| IBIS file imx8dxl_15x15_rev1_15.ibs generated by Viper version: 2018.06.11
[IBIS Ver]   5.1
[Comment Char]   |_char
[File Name]   imx8dxl_15x15_rev1_15.ibs
[File Rev]   1.15
[Date]   Mon Sep  2 11:08:28 2019
[Source]   NXP Viper 2018.06.11
[Notes]
   Warning 'pullup_ref' Exceeds 15 characters: VDD_PCIE_DIG_1P8_3P3 was cut to VDD_PCIE_DIG_1P
   Warning 'pullup_ref' Exceeds 15 characters: VDD_PCIE_LDO_1P0_CAP was cut to VDD_PCIE_LDO_1P
   Warning 'pullup_ref' Exceeds 15 characters: VDD_EMMC0_1P8_3P3 was cut to VDD_EMMC0_1P8_3
   Warning 'pullup_ref' Exceeds 15 characters: VDD_USDHC1_VSELECT_1P8_3P3 was cut to VDD_USDHC1_VSEL
   Warning 'pullup_ref' Exceeds 15 characters: VDD_ENET0_1P8_3P3 was cut to VDD_ENET0_1P8_3
   Warning 'pullup_ref' Exceeds 15 characters: VDD_ENET0_VSELECT_1P8_3P3 was cut to VDD_ENET0_VSELE
   Warning 'pullup_ref' Exceeds 15 characters: VDD_ENET_MDIO_1P8_3P3 was cut to VDD_ENET_MDIO_1
   Warning 'pullup_ref' Exceeds 15 characters: VDD_ESAI_SPDIF_1P8_3P3 was cut to VDD_ESAI_SPDIF_
   Warning 'pullup_ref' Exceeds 15 characters: VDD_SPI_MCLK_UART_1P8_3P3 was cut to VDD_SPI_MCLK_UA
   Warning 'pullup_ref' Exceeds 15 characters: VDD_SPI_SAI_1P8_3P3 was cut to VDD_SPI_SAI_1P8
   Warning 'pullup_ref' Exceeds 15 characters: VDD_QSPI0B_1P8_3P3 was cut to VDD_QSPI0B_1P8_
   Warning 'pullup_ref' Exceeds 15 characters: VDD_QSPI0A_1P8_3P3 was cut to VDD_QSPI0A_1P8_
   Warning 'pullup_ref' Exceeds 15 characters: VDD_TMPR_CSI_1P8_3P3 was cut to VDD_TMPR_CSI_1P
   Warning 'pullup_ref' Exceeds 15 characters: VDD_SNVS_LDO_1P8_CAP was cut to VDD_SNVS_LDO_1P
   Warning 'pullup_ref' Exceeds 15 characters: VDD_CAN_UART_1P8_3P3 was cut to VDD_CAN_UART_1P
[Disclaimer] IMPORTANT NOTICE
  This information is provided on an AS IS basis and without warranty.
  IN NO EVENT SHALL NXP BE LIABLE FOR INCIDENTAL OR CONSEQUENTIAL
  DAMAGES ARISING FROM USE OF THIS INFORMATION. THIS DISCLAIMER OF
  WARRANTY EXTENDS TO THE USER OF THE INFORMATION, AND TO THEIR CUSTOMERS
  OR USERS OF PRODUCTS  AND IS IN LIEU OF ALL WARRANTIES WHETHER EXPRESS,
  IMPLIED, OR STATUTORY, INCLUDING IMPLIED WARRANTIES OF MERCHANTABILITY
  OR FITNESS FOR PARTICULAR PURPOSE.
  NXP does not represent or warrant that the information furnished
  hereunder is free of infringement of any third party patents,
  copyrights, trade secrets, or other intellectual property rights.
  NXP does not represent or warrant that the information is free of
  defect, or that it meets any particular standard, requirements or need
  of the user of the infomation or their customers.
  NXP reserves the right to change the information in this file
  without notice.
   http://www.nxp.com
[Copyright]   (C) Copyright NXP 2004 - 2019, All Rights Reserved.
|   15x15
[Component]   15x15
[Manufacturer]   NXP
[Package]
| variable   typ   min   max
R_pkg   0.39888   0.071395   0.70153
L_pkg   2.436e-09   7.469e-10   4.204e-09
C_pkg   1.081e-12   6.841e-13   1.885e-12
[Pin] signal_name   model_name   R_pin   L_pin   C_pin
A1   VSS_MAIN   GND   NA   NA   NA
A3   DDR_DCF22   PDDRIO_PAD_COMMAND   0.69334   4.204e-09 1.534e-12
A5   DDR_DCF09   PDDRIO_PAD_COMMAND   0.65039   4.090e-09 1.750e-12
A7   DDR_DCF04   PDDRIO_PAD_COMMAND   0.70153   4.051e-09 1.549e-12
A9   PCIE_CTRL0_WAKE_B   BDPROGSCARUDQP_SDMMC_STD_3V3SF_FC_OUTER  0.37798   2.410e-09 9.804e-13
A11   PCIE0_TX0_P   ABI_SERDES   0.33546   2.531e-09 1.007e-12
A13   PCIE0_RX0_P   ABI_SERDES   0.33039   2.526e-09 1.001e-12
A15   PCIE_REFCLK100M_P   NC   0.39132   2.612e-09 9.561e-13
A17   USB_OTG2_DP   USB2_NXP   0.36476   2.455e-09 9.409e-13
A19   USB_OTG1_DN   USB2_NXP   0.3104   2.238e-09 9.070e-13
A21   EMMC0_DATA7   BDPROGSCARUDQP_SDMMC_STD_3V3SF_FC_OUTER  0.50159   3.076e-09 1.290e-12
A23   EMMC0_DATA0   BDPROGSCARUDQP_SDMMC_STD_3V3SF_FC_INNER  0.39707   2.449e-09 1.054e-12
A25   EMMC0_DATA5   BDPROGSCARUDQP_SDMMC_STD_3V3SF_FC_OUTER  0.39485   2.459e-09 1.043e-12
A27   EMMC0_CMD   BDPROGSCARUDQP_SDMMC_STD_3V3SF_FC_OUTER  0.47205   2.883e-09 1.198e-12
A29   USDHC1_RESET_B   BDPROGSCARUDQP_SDMMC_STD_3V3SF_FC_INNER  0.43085   2.711e-09 1.176e-12
A31   ENET0_RGMII_RXD3   BDPROGSCARUDQP_SDMMC_STD_3V3SF_FC_OUTER  0.5841   3.378e-09 1.362e-12
A33   ENET0_RGMII_RXD1   BDPROGSCARUDQP_SDMMC_STD_3V3SF_FC_OUTER  0.49079   2.887e-09 1.171e-12
A35   VSS_MAIN   GND   NA   NA   NA
B2   DDR_DCF20   PDDRIO_PAD_COMMAND   0.63836   3.791e-09 1.427e-12
B4   DDR_DCF17   PDDRIO_PAD_COMMAND   0.58041   3.372e-09 1.383e-12
B6   DDR_DCF19   PDDRIO_PAD_COMMAND   0.63149   3.649e-09 1.445e-12
B8   PCIE_CTRL0_PERST_B   BDPROGSCARUDQP_SDMMC_STD_3V3SF_FC_OUTER  0.32639   2.064e-09 1.009e-12
B10   PCIE0_TX0_N   ABI_SERDES   0.34946   2.450e-09 1.035e-12
B12   PCIE0_RX0_N   ABI_SERDES   0.33887   2.428e-09 1.004e-12
B14   PCIE_REFCLK100M_N   NC   0.39474   2.595e-09 9.576e-13
B16   USB_OTG2_DN   USB2_NXP   0.35865   2.350e-09 9.326e-13
B18   USB_OTG1_DP   USB2_NXP   0.32362   2.267e-09 9.280e-13
B20   EMMC0_DATA6   BDPROGSCARUDQP_SDMMC_STD_3V3SF_FC_INNER  0.34554   2.183e-09 9.968e-13
B22   EMMC0_DATA1   BDPROGSCARUDQP_SDMMC_STD_3V3SF_FC_OUTER  0.31728   1.984e-09 9.313e-13
B24   EMMC0_DATA3   BDPROGSCARUDQP_SDMMC_STD_3V3SF_FC_OUTER  0.32903   2.044e-09 9.577e-13
B26   EMMC0_RESET_B   BDPROGSCARUDQP_SDMMC_STD_3V3SF_FC_OUTER  0.37344   2.349e-09 1.036e-12
B28   USDHC1_VSELECT   BDPROGSCARUDQP_SDMMC_STD_3V3SF_FC_OUTER  0.43171   2.674e-09 1.183e-12
B30   USDHC1_WP   BDPROGSCARUDQP_SDMMC_STD_3V3SF_FC_INNER  0.43147   2.643e-09 1.163e-12
B32   ENET0_RGMII_RXD0   BDPROGSCARUDQP_SDMMC_STD_3V3SF_FC_INNER  0.49885   2.934e-09 1.197e-12
B34   ENET0_RGMII_RXC   BDPROGSCARUDQP_SDMMC_STD_3V3SF_FC_INNER  0.52236   3.036e-09 1.292e-12
C1   VSS_MAIN   GND   NA   NA   NA
C3   VSS_MAIN   GND   NA   NA   NA
C5   DDR_DCF32   PDDRIO_PAD_COMMAND   0.42657   2.729e-09 1.182e-12
C7   VSS_MAIN   GND   NA   NA   NA
C9   PCIE_CTRL0_CLKREQ_B   BDPROGSCARUDQP_SDMMC_STD_3V3SF_FC_INNER  0.31061   1.972e-09 8.875e-13
C11   VSS_MAIN   GND   NA   NA   NA
C13   VSS_MAIN   GND   NA   NA   NA
C15   VSS_MAIN   GND   NA   NA   NA
C17   VSS_MAIN   GND   NA   NA   NA
C19   USB_OTG1_ID   NC   0.32886   2.060e-09 9.688e-13
C21   EMMC0_DATA2   BDPROGSCARUDQP_SDMMC_STD_3V3SF_FC_INNER  0.28685   1.796e-09 8.761e-13
C23   EMMC0_DATA4   BDPROGSCARUDQP_SDMMC_STD_3V3SF_FC_INNER  0.28187   1.779e-09 8.664e-13
C25   EMMC0_STROBE   BDPROGSCARUDQP_SDMMC_STD_3V3SF_FC_INNER  0.33656   2.067e-09 9.738e-13
C27   EMMC0_CLK   BDPROGSCARUDQP_SDMMC_STD_3V3SF_FC_INNER  0.52053   3.084e-09 1.318e-12
C29   USDHC1_CD_B   BDPROGSCARUDQP_SDMMC_STD_3V3SF_FC_OUTER  0.42428   2.608e-09 1.152e-12
C31   ENET0_RGMII_RXD2   BDPROGSCARUDQP_SDMMC_STD_3V3SF_FC_INNER  0.52682   3.001e-09 1.274e-12
C33   ENET0_RGMII_RX_CTL   BDPROGSCARUDQP_SDMMC_STD_3V3SF_FC_OUTER  0.42005   2.537e-09 1.127e-12
C35   ENET0_RGMII_TX_CTL   BDPROGSCARUDQP_SDMMC_STD_3V3SF_FC_OUTER  0.51478   3.058e-09 1.280e-12
D2   VSS_MAIN   GND   NA   NA   NA
D34   ENET0_REFCLK_125M_25M   BDPROGSCARUDQP_SDMMC_STD_3V3SF_FC_OUTER  0.45684   2.681e-09 1.102e-12
E1   DDR_DCF24   PDDRIO_PAD_COMMAND   0.6095   3.695e-09 1.338e-12
E3   DDR_DCF27   PDDRIO_PAD_COMMAND   0.43126   2.639e-09 1.204e-12
E5   VSS_MAIN   GND   NA   NA   NA
E7   VSS_MAIN   GND   NA   NA   NA
E9   VSS_MAIN   GND   NA   NA   NA
E11   VDD_PCIE_LDO_1P0_CAP   POWER   NA   NA   NA
E13   VSS_MAIN   GND   NA   NA   NA
E15   VDD_ANA0_1P8   POWER   NA   NA   NA
E17   VSS_MAIN   GND   NA   NA   NA
E19   VSS_MAIN   GND   NA   NA   NA
E21   VSS_MAIN   GND   NA   NA   NA
E23   VSS_MAIN   GND   NA   NA   NA
E25   VSS_MAIN   GND   NA   NA   NA
E27   VSS_MAIN   GND   NA   NA   NA
E29   VSS_MAIN   GND   NA   NA   NA
E31   VSS_MAIN   GND   NA   NA   NA
E33   ENET0_MDC   BDPROGSCARUDQP_SDMMC_STD_3V3SF_FC_OUTER  0.39205   2.311e-09 1.041e-12
E35   ENET0_MDIO   BDPROGSCARUDQP_SDMMC_STD_3V3SF_FC_INNER  0.47347   2.857e-09 1.148e-12
F2   DDR_DCF23   PDDRIO_PAD_COMMAND   0.51126   3.016e-09 1.214e-12
F34   ENET1_RGMII_RXD1   BDPROGSCARUDQP_SDMMC_STD_3V3SF_FC_OUTER  0.46877   2.793e-09 1.175e-12
G1   DDR_DCF26   PDDRIO_PAD_COMMAND   0.5185   3.175e-09 1.322e-12
G3   VSS_MAIN   GND   NA   NA   NA
G5   VSS_MAIN   GND   NA   NA   NA
G9   PCIE_REXT   NC   0.34925   2.509e-09 1.529e-12
G11   PCIE_REF_QR   NC   0.23973   1.816e-09 9.243e-13
G13   USB_OTG2_VBUS   hs_vbus_input   0.21475   1.509e-09 7.043e-13
G15   USB_OTG2_ID   NC   0.21462   1.402e-09 7.583e-13
G17   USB_OTG1_VBUS   hs_vbus_input   0.24172   1.565e-09 7.717e-13
G19   USB_SS3_TC1   BDPROGSCARUDQP_SDMMC_STD_3V3SF_FC_OUTER  0.19904   1.304e-09 6.960e-13
G21   USB_SS3_TC0   BDPROGSCARUDQP_SDMMC_STD_3V3SF_FC_INNER  0.30844   1.974e-09 9.084e-13
G23   USB_SS3_TC3   BDPROGSCARUDQP_SDMMC_STD_3V3SF_FC_OUTER  0.29844   1.856e-09 9.049e-13
G25   USB_SS3_TC2   BDPROGSCARUDQP_SDMMC_STD_3V3SF_FC_INNER  0.40848   2.503e-09 1.109e-12
G27   ENET0_RGMII_TXC   BDPROGSCARUDQP_SDMMC_STD_3V3SF_FC_INNER  0.24271   1.576e-09 8.194e-13
G29   ENET0_RGMII_TXD1   BDPROGSCARUDQP_SDMMC_STD_3V3SF_FC_OUTER  0.3428   2.080e-09 9.846e-13
G31   VSS_MAIN   GND   NA   NA   NA
G33   ENET1_RGMII_RXC   BDPROGSCARUDQP_SDMMC_STD_3V3SF_FC_INNER  0.39056   2.383e-09 1.023e-12
G35   ENET1_RGMII_RXD3   BDPROGSCARUDQP_SDMMC_STD_3V3SF_FC_OUTER  0.44701   2.719e-09 1.173e-12
H2   DDR_DCF18   PCKE_PAD   0.49331   2.908e-09 1.114e-12
H34   ENET1_RGMII_RXD2   BDPROGSCARUDQP_SDMMC_STD_3V3SF_FC_INNER  0.40015   2.450e-09 1.063e-12
J1   DDR_DCF01   PDDRIO_PAD_COMMAND   0.54249   3.171e-09 1.259e-12
J3   DDR_DCF03   PDDRIO_PAD_COMMAND   0.49918   2.845e-09 1.237e-12
J5   VSS_MAIN   GND   NA   NA   NA
J7   DDR_DCF28   PDDRIO_PAD_COMMAND   0.27786   1.824e-09 8.557e-13
J9   DDR_DCF33   PDDRIO_PAD_COMMAND   0.37754   2.473e-09 1.129e-12
J11   PCIE0_PHY_PLL_REF_RETURN   GND   0.071395  7.469e-10 1.106e-12
J13   VDD_PCIE_1P8   POWER   NA   NA   NA
J17   VDD_USB_SS3_LDO_1P0_CAP   POWER   NA   NA   NA
J19   VDD_USB_1P8   POWER   NA   NA   NA
J21   VDD_USB_3P3   POWER   NA   NA   NA
J23   VDD_EMMC0_1P8_3P3   POWER   NA   NA   NA
J25   VDD_EMMC0_1P8_3P3   POWER   NA   NA   NA
J27   VDD_USDHC1_VSELECT_1P8_3P3   POWER   NA   NA   NA
J29   ENET0_RGMII_TXD0   BDPROGSCARUDQP_SDMMC_STD_3V3SF_FC_INNER  0.36245   2.190e-09 9.561e-13
J31   VSS_MAIN   GND   NA   NA   NA
J33   ENET1_RGMII_RXD0   BDPROGSCARUDQP_SDMMC_STD_3V3SF_FC_INNER  0.39699   2.409e-09 1.053e-12
J35   ENET1_RGMII_RX_CTL   BDPROGSCARUDQP_SDMMC_STD_3V3SF_FC_OUTER  0.46113   2.750e-09 1.160e-12
K2   DDR_CK0_N   PCK_PAD   0.59967   3.394e-09 1.352e-12
K34   ENET1_REFCLK_125M_25M   BDPROGSCARUDQP_SDMMC_STD_3V3SF_FC_OUTER  0.40652   2.458e-09 1.069e-12
L1   DDR_CK0_P   PCK_PAD   0.58582   3.373e-09 1.364e-12
L3   VSS_MAIN   GND   NA   NA   NA
L5   VSS_MAIN   GND   NA   NA   NA
L7   DDR_DCF30   PCKE_PAD   0.27406   1.691e-09 8.614e-13
L9   VDD_PCIE_DIG_1P8_3P3   POWER   NA   NA   NA
L11   VSS_MAIN   GND   NA   NA   NA
L13   VSS_MAIN   GND   NA   NA   NA
L15   VSS_MAIN   GND   NA   NA   NA
L17   VSS_MAIN   GND   NA   NA   NA
L19   VSS_MAIN   GND   NA   NA   NA
L21   VSS_MAIN   GND   NA   NA   NA
L23   VSS_MAIN   GND   NA   NA   NA
L25   VSS_MAIN   GND   NA   NA   NA
L27   VDD_ENET0_VSELECT_1P8_3P3   POWER   NA   NA   NA
L29   ENET0_RGMII_TXD2   BDPROGSCARUDQP_SDMMC_STD_3V3SF_FC_INNER  0.3233   2.047e-09 9.997e-13
L31   VSS_MAIN   GND   NA   NA   NA
L33   ENET1_RGMII_TXD3   BDPROGSCARUDQP_SDMMC_STD_3V3SF_FC_OUTER  0.35635   2.156e-09 9.575e-13
L35   ENET1_RGMII_TXC   BDPROGSCARUDQP_SDMMC_STD_3V3SF_FC_INNER  0.5103   3.102e-09 1.230e-12
M2   DDR_DCF05   PDDRIO_PAD_COMMAND   0.3749   2.205e-09 9.777e-13
M34   ENET1_RGMII_TXD2   BDPROGSCARUDQP_SDMMC_STD_3V3SF_FC_OUTER  0.52172   3.043e-09 1.266e-12
N1   DDR_DCF00   PDDRIO_PAD_COMMAND   0.39316   2.320e-09 1.064e-12
N3   DDR_DCF08   PDDRIO_PAD_COMMAND   0.51713   2.935e-09 1.237e-12
N5   VSS_MAIN   GND   NA   NA   NA
N7   VDD_DDR_VDDQ   POWER   NA   NA   NA
N9   VDD_DDR_VDDQ   POWER   NA   NA   NA
N11   VSS_MAIN   GND   NA   NA   NA
N13   VDD_MEMC   POWER   NA   NA   NA
N15   VDD_MAIN   POWER   NA   NA   NA
N17   VDD_MAIN   POWER   NA   NA   NA
N19   VDD_MAIN   POWER   NA   NA   NA
N21   VDD_MAIN   POWER   NA   NA   NA
N23   VDD_MAIN   POWER   NA   NA   NA
N25   VSS_MAIN   GND   NA   NA   NA
N27   VDD_ENET0_1P8_3P3   POWER   NA   NA   NA
N29   ENET0_RGMII_TXD3   BDPROGSCARUDQP_SDMMC_STD_3V3SF_FC_OUTER  0.33799   2.054e-09 9.689e-13
N31   VSS_MAIN   GND   NA   NA   NA
N33   ENET1_RGMII_TXD0   BDPROGSCARUDQP_SDMMC_STD_3V3SF_FC_INNER  0.37304   2.268e-09 1.025e-12
N35   ENET1_RGMII_TXD1   BDPROGSCARUDQP_SDMMC_STD_3V3SF_FC_OUTER  0.43036   2.644e-09 1.159e-12
P2   DDR_DCF15   PCKE_PAD   0.44408   2.646e-09 1.078e-12
P34   SPI3_SCK   BDPROGSCARUDQP_SDMMC_STD_3V3SF_FC_INNER  0.34281   2.124e-09 9.884e-13
R1   DDR_DCF10   PDDRIO_PAD_COMMAND   0.47803   2.820e-09 1.199e-12
R3   VSS_MAIN   GND   NA   NA   NA
R5   VSS_MAIN   GND   NA   NA   NA
R7   VDD_DDR_VDDQ   POWER   NA   NA   NA
R9   VDD_DDR_VDDQ   POWER   NA   NA   NA
R11   VSS_MAIN   GND   NA   NA   NA
R13   VDD_MEMC   POWER   NA   NA   NA
R15   VDD_MAIN   POWER   NA   NA   NA
R17   VDD_MAIN   POWER   NA   NA   NA
R19   VSS_MAIN   GND   NA   NA   NA
R21   VSS_MAIN   GND   NA   NA   NA
R23   VDD_MAIN   POWER   NA   NA   NA
R25   VSS_MAIN   GND   NA   NA   NA
R27   VDD_ENET_MDIO_1P8_3P3   POWER   NA   NA   NA
R29   ENET1_RGMII_TX_CTL   BDPROGSCARUDQP_SDMMC_STD_3V3SF_FC_INNER  0.40442   2.374e-09 1.066e-12
R31   VSS_MAIN   GND   NA   NA   NA
R33   SPI3_SDI   BDPROGSCARUDQP_SDMMC_STD_3V3SF_FC_INNER  0.34862   2.106e-09 9.636e-13
R35   SPI3_SDO   BDPROGSCARUDQP_SDMMC_STD_3V3SF_FC_OUTER  0.41808   2.511e-09 1.122e-12
T2   DDR_DCF14   PCKE_PAD   0.41078   2.375e-09 9.867e-13
T34   SPI3_CS0   BDPROGSCARUDQP_SDMMC_STD_3V3SF_FC_OUTER  0.36788   2.237e-09 1.022e-12
U1   DDR_DCF16   PDDRIO_PAD_COMMAND   0.37334   2.217e-09 8.753e-13
U3   DDR_DCF12   PDDRIO_PAD_COMMAND   0.37509   2.173e-09 9.658e-13
U5   VSS_MAIN   GND   NA   NA   NA
U7   VDD_DDR_VDDQ   POWER   NA   NA   NA
U9   VDD_DDR_VDDQ   POWER   NA   NA   NA
U11   VSS_MAIN   GND   NA   NA   NA
U13   VDD_MEMC   POWER   NA   NA   NA
U15   VSS_MAIN   GND   NA   NA   NA
U17   VSS_MAIN   GND   NA   NA   NA
U19   VDD_MEMC   POWER   NA   NA   NA
U21   VSS_MAIN   GND   NA   NA   NA
U23   VDD_MAIN   POWER   NA   NA   NA
U25   VSS_MAIN   GND   NA   NA   NA
U27   VDD_ESAI_SPDIF_1P8_3P3   POWER   NA   NA   NA
U29   SPI3_CS1   BDPROGSCARUDQP_SDMMC_STD_3V3SF_FC_INNER  0.27919   1.718e-09 8.422e-13
U31   VSS_MAIN   GND   NA   NA   NA
U33   MCLK_IN0   BDPROGSCARUDQP_SDMMC_STD_3V3SF_FC_INNER  0.28929   1.788e-09 8.790e-13
U35   MCLK_IN1   BDPROGSCARUDQP_SDMMC_STD_3V3SF_FC_OUTER  0.37626   2.307e-09 1.050e-12
V2   DDR_DCF21   PDDRIO_PAD_COMMAND   0.48159   2.850e-09 1.140e-12
V34   MCLK_OUT0   BDPROGSCARUDQP_SDMMC_STD_3V3SF_FC_OUTER  0.36526   2.211e-09 9.998e-13
W1   DDR_DCF11   PDDRIO_PAD_COMMAND   0.40855   2.365e-09 9.927e-13
W3   VSS_MAIN   GND   NA   NA   NA
W5   VSS_MAIN   GND   NA   NA   NA
W7   VDD_DDR_PLL_1P8   POWER   NA   NA   NA
W9   VDD_DDR_VDDQ   POWER   NA   NA   NA
W11   VSS_MAIN   GND   NA   NA   NA
W13   VDD_MEMC   POWER   NA   NA   NA
W15   VDD_MEMC   POWER   NA   NA   NA
W17   VDD_MEMC   POWER   NA   NA   NA
W19   VDD_MEMC   POWER   NA   NA   NA
W21   VSS_MAIN   GND   NA   NA   NA
W23   VDD_MAIN   POWER   NA   NA   NA
W25   VSS_MAIN   GND   NA   NA   NA
W27   VDD_SPI_MCLK_UART_1P8_3P3   POWER   NA   NA   NA
W29   UART1_RTS_B   BDPROGSCARUDQP_SDMMC_STD_3V3SF_FC_INNER  0.1996   1.313e-09 6.989e-13
W31   VSS_MAIN   GND   NA   NA   NA
W33   UART1_RX   BDPROGSCARUDQP_SDMMC_STD_3V3SF_FC_OUTER  0.28697   1.794e-09 8.407e-13
W35   UART1_TX   BDPROGSCARUDQP_SDMMC_STD_3V3SF_FC_INNER  0.37477   2.324e-09 1.012e-12
Y2   DDR_DCF07   PDDRIO_PAD_COMMAND   0.54086   3.096e-09 1.259e-12
Y34   SPI0_SCK   BDPROGSCARUDQP_SDMMC_STD_3V3SF_FC_OUTER  0.34397   2.096e-09 1.004e-12
AA1   DDR_DQ14   PDDRIO_PAD_DATA   0.38686   2.266e-09 1.007e-12
AA3   DDR_DQ15   PDDRIO_PAD_DATA   0.37106   2.106e-09 9.193e-13
AA5   VSS_MAIN   GND   NA   NA   NA
AA7   VDD_DDR_VDDQ   POWER   NA   NA   NA
AA9   VDD_DDR_VDDQ   POWER   NA   NA   NA
AA11  VSS_MAIN   GND   NA   NA   NA
AA13  VDD_MEMC   POWER   NA   NA   NA
AA15  VSS_MAIN   GND   NA   NA   NA
AA17  VSS_MAIN   GND   NA   NA   NA
AA19  VSS_MAIN   GND   NA   NA   NA
AA21  VSS_MAIN   GND   NA   NA   NA
AA23  VDD_MAIN   POWER   NA   NA   NA
AA25  VSS_MAIN   GND   NA   NA   NA
AA27  VDD_SPI_SAI_1P8_3P3   POWER   NA   NA   NA
AA29  UART1_CTS_B   BDPROGSCARUDQP_SDMMC_STD_3V3SF_FC_OUTER  0.30711   1.850e-09 8.984e-13
AA31  VSS_MAIN   GND   NA   NA   NA
AA33  SPI0_SDI   BDPROGSCARUDQP_SDMMC_STD_3V3SF_FC_INNER  0.30864   1.887e-09 8.853e-13
AA35  SPI0_SDO   BDPROGSCARUDQP_SDMMC_STD_3V3SF_FC_OUTER  0.38081   2.323e-09 1.024e-12
AB2   DDR_DQ13   PDDRIO_PAD_DATA   0.39469   2.222e-09 9.773e-13
AB34  SPI0_CS0   BDPROGSCARUDQP_SDMMC_STD_3V3SF_FC_OUTER  0.35488   2.169e-09 1.015e-12
AC1   DDR_DQ12   PDDRIO_PAD_DATA   0.38503   2.238e-09 1.020e-12
AC3   VSS_MAIN   GND   NA   NA   NA
AC5   VSS_MAIN   GND   NA   NA   NA
AC7   DDR_ATO   NC   0.32348   2.050e-09 9.221e-13
AC9   VDD_DDR_VDDQ   POWER   NA   NA   NA
AC11  VSS_MAIN   GND   NA   NA   NA
AC13  VDD_MEMC   POWER   NA   NA   NA
AC15  VDD_MEMC   POWER   NA   NA   NA
AC17  VDD_MAIN   POWER   NA   NA   NA
AC19  VDD_MAIN   POWER   NA   NA   NA
AC21  VDD_MAIN   POWER   NA   NA   NA
AC23  VDD_MAIN   POWER   NA   NA   NA
AC25  VSS_MAIN   GND   NA   NA   NA
AC27  VDD_ADC_1P8   POWER   NA   NA   NA
AC29  ADC_VREFH   POWER   0.17517   1.349e-09 1.175e-12
AC31  VSS_MAIN   GND   NA   NA   NA
AC33  ADC_IN2   BDPROGSCRUDQP_EXT_CSF_1V8_FC_OUTER   0.32371   1.993e-09 9.156e-13
AC35  SPI0_CS1   BDPROGSCARUDQP_SDMMC_STD_3V3SF_FC_INNER  0.41744   2.490e-09 1.124e-12
AD2   DDR_DQS1_N   PDQS_PAD   0.41624   2.445e-09 9.848e-13
AD34  ADC_IN0   BDPROGSCRUDQP_EXT_CSF_1V8_FC_OUTER   0.3697   2.251e-09 1.027e-12
AE1   DDR_DM1   PDDRIO_PAD_DATA   0.4081   2.366e-09 1.047e-12
AE3   DDR_DQS1_P   PDQS_PAD   0.39825   2.300e-09 9.964e-13
AE5   VSS_MAIN   GND   NA   NA   NA
AE7   VDD_DDR_VDDQ   POWER   NA   NA   NA
AE9   VDD_DDR_VDDQ   POWER   NA   NA   NA
AE11  VSS_MAIN   GND   NA   NA   NA
AE13  VSS_MAIN   GND   NA   NA   NA
AE15  VSS_MAIN   GND   NA   NA   NA
AE17  VSS_MAIN   GND   NA   NA   NA
AE19  VSS_MAIN   GND   NA   NA   NA
AE21  VSS_MAIN   GND   NA   NA   NA
AE23  VSS_MAIN   GND   NA   NA   NA
AE25  VSS_MAIN   GND   NA   NA   NA
AE27  VDD_ADC_DIG_1P8   POWER   NA   NA   NA
AE29  ADC_VREFL   GND   0.18668   1.456e-09 1.351e-12
AE31  VSS_MAIN   GND   NA   NA   NA
AE33  ADC_IN4   BDPROGSCRUDQP_EXT_CSF_1V8_FC_OUTER   0.30466   1.915e-09 9.342e-13
AE35  ADC_IN1   BDPROGSCRUDQP_EXT_CSF_1V8_FC_INNER   0.40353   2.468e-09 1.104e-12
AF2   DDR_DQ11   PDDRIO_PAD_DATA   0.44062   2.642e-09 1.018e-12
AF34  ADC_IN3   BDPROGSCRUDQP_EXT_CSF_1V8_FC_INNER   0.42653   2.545e-09 1.146e-12
AG1   DDR_DQ10   PDDRIO_PAD_DATA   0.43352   2.579e-09 1.081e-12
AG3   VSS_MAIN   GND   NA   NA   NA
AG5   VSS_MAIN   GND   NA   NA   NA
AG7   DDR_DTO0   PDDRIO_PAD_COMMAND   0.5282   2.985e-09 1.211e-12
AG9   DDR_DTO1   PDDRIO_PAD_COMMAND   0.55162   3.295e-09 1.339e-12
AG11  VDD_QSPI0B_1P8_3P3   POWER   NA   NA   NA
AG13  VDD_QSPI0A_1P8_3P3   POWER   NA   NA   NA
AG15  VDD_CSI_1P8_3P3   POWER   NA   NA   NA
AG17  VDD_TMPR_CSI_1P8_3P3   POWER   NA   NA   NA
AG19  VDD_SNVS_LDO_1P8_CAP   POWER   NA   NA   NA
AG21  VDD_SNVS_4P2   NC   NA   NA   NA
AG23  RTC_XTALI   NC   0.21145   1.418e-09 7.113e-13
AG25  XTALI   NC   0.23031   1.470e-09 7.628e-13
AG27  VDD_CAN_UART_1P8_3P3   POWER   NA   NA   NA
AG29  JTAG_TRST_B   BDPROGSCRUDQP_EXT_CSF_1V8_FC_INNER   0.28217   1.721e-09 8.060e-13
AG31  VSS_MAIN   GND   NA   NA   NA
AG33  VSS_MAIN   GND   NA   NA   NA
AG35  ADC_IN5   BDPROGSCRUDQP_EXT_CSF_1V8_FC_INNER   0.41989   2.578e-09 1.105e-12
AH2   DDR_DQ09   PDDRIO_PAD_DATA   0.47494   2.829e-09 1.093e-12
AH34  FLEXCAN0_RX   BDPROGSCARUDQP_SDMMC_STD_3V3SF_FC_INNER  0.41655   2.468e-09 1.086e-12
AJ1   DDR_DQ00   PDDRIO_PAD_DATA   0.46352   2.784e-09 1.086e-12
AJ3   DDR_DQ08   PDDRIO_PAD_DATA   0.43935   2.551e-09 1.100e-12
AJ5   VSS_MAIN   GND   NA   NA   NA
AJ7   DDR_ZQ   NC   0.3021   2.142e-09 1.570e-12
AJ9   DDR_VREF   NC   0.096523  1.237e-09 1.885e-12
AJ11  QSPI0B_SS0_B   BDPROGSCARUDQP_SDMMC_STD_3V3SF_FC_OUTER  0.24419   1.567e-09 8.053e-13
AJ13  SNVS_TAMPER_IN4   NC   0.38351   2.338e-09 1.070e-12
AJ15  SNVS_TAMPER_IN3   NC   0.20743   1.385e-09 7.258e-13
AJ17  SNVS_TAMPER_IN2   NC   0.21744   1.420e-09 7.260e-13
AJ19  ANA_TEST_OUT_P   NC   0.39807   2.428e-09 1.126e-12
AJ21  ANA_TEST_OUT_N   NC   0.40158   2.410e-09 1.122e-12
AJ23  RTC_XTALO   NC   0.19645   1.274e-09 6.841e-13
AJ25  XTALO   NC   0.21772   1.406e-09 7.147e-13
AJ27  VDD_ANA1_1P8   POWER   NA   NA   NA
AJ29  SCU_BOOT_MODE2   BDPROGSCRUDQP_EXT_CSF_1V8_FC_OUTER   0.12342   1.725e-09 1.190e-12
AJ31  VSS_MAIN   GND   NA   NA   NA
AJ33  FLEXCAN1_RX   BDPROGSCARUDQP_SDMMC_STD_3V3SF_FC_INNER  0.43258   2.531e-09 1.154e-12
AJ35  FLEXCAN0_TX   BDPROGSCARUDQP_SDMMC_STD_3V3SF_FC_OUTER  0.43771   2.647e-09 1.127e-12
AK2   DDR_DQ01   PDDRIO_PAD_DATA   0.46167   2.644e-09 1.154e-12
AK34  FLEXCAN1_TX   BDPROGSCARUDQP_SDMMC_STD_3V3SF_FC_OUTER  0.44184   2.635e-09 1.191e-12
AL1   DDR_DQ02   PDDRIO_PAD_DATA   0.53669   3.200e-09 1.206e-12
AL3   VSS_MAIN   GND   NA   NA   NA
AL5   VSS_MAIN   GND   NA   NA   NA
AL7   VSS_MAIN   GND   NA   NA   NA
AL9   VSS_MAIN   GND   NA   NA   NA
AL11  VSS_MAIN   GND   NA   NA   NA
AL13  VSS_MAIN   GND   NA   NA   NA
AL15  VSS_MAIN   GND   NA   NA   NA
AL17  VSS_MAIN   GND   NA   NA   NA
AL19  VSS_MAIN   GND   NA   NA   NA
AL21  VSS_MAIN   GND   NA   NA   NA
AL23  VSS_MAIN   GND   NA   NA   NA
AL25  VSS_MAIN   GND   NA   NA   NA
AL27  VSS_MAIN   GND   NA   NA   NA
AL29  VSS_MAIN   GND   NA   NA   NA
AL31  VSS_MAIN   GND   NA   NA   NA
AL33  FLEXCAN2_TX   BDPROGSCARUDQP_SDMMC_STD_3V3SF_FC_OUTER  0.45601   2.680e-09 1.152e-12
AL35  FLEXCAN2_RX   BDPROGSCARUDQP_SDMMC_STD_3V3SF_FC_INNER  0.48944   2.922e-09 1.193e-12
AM2   DDR_DQ03   PDDRIO_PAD_DATA   0.46409   2.669e-09 1.182e-12
AM34  UART0_RX   BDPROGSCARUDQP_SDMMC_STD_3V3SF_FC_INNER  0.47763   2.805e-09 1.193e-12
AN1   DDR_DQS0_P   PDQS_PAD   0.6104   3.546e-09 1.363e-12
AN3   DDR_DM0   PDDRIO_PAD_DATA   0.42725   2.515e-09 1.098e-12
AN5   VSS_MAIN   GND   NA   NA   NA
AN7   QSPI0A_SS0_B   BDPROGSCARUDQP_SDMMC_STD_3V3SF_FC_OUTER  0.37675   2.298e-09 1.048e-12
AN9   QSPI0A_DATA2   BDPROGSCARUDQP_SDMMC_STD_3V3SF_FC_INNER  0.38375   2.311e-09 1.052e-12
AN11  QSPI0A_DATA3   BDPROGSCARUDQP_SDMMC_STD_3V3SF_FC_OUTER  0.34178   2.086e-09 9.216e-13
AN13  QSPI0A_DATA1   BDPROGSCARUDQP_SDMMC_STD_3V3SF_FC_OUTER  0.2945   1.842e-09 8.556e-13
AN15  QSPI0B_DQS   BDPROGSCARUDQP_SDMMC_STD_3V3SF_FC_OUTER  0.3697   2.292e-09 1.025e-12
AN17  SNVS_TAMPER_IN1   NC   0.27993   1.762e-09 8.480e-13
AN19  SNVS_TAMPER_IN0   NC   0.27957   1.750e-09 8.625e-13
AN21  SNVS_TAMPER_OUT2   NC   0.30845   1.951e-09 9.145e-13
AN23  SNVS_TAMPER_OUT4   NC   0.33912   2.092e-09 9.936e-13
AN25  SCU_PMIC_STANDBY   BDPROGSCRUDQP_EXT_CSF_1V8_FC_INNER   0.39664   2.362e-09 1.048e-12
AN27  PMIC_INT_B   BDPROGSCRUDQP_EXT_CSF_1V8_FC_OUTER   0.38604   2.361e-09 1.073e-12
AN29  TEST_MODE_SELECT   BDPROGSCRUDQP_EXT_CSF_1V8_FC_OUTER   0.43855   2.521e-09 1.093e-12
AN31  JTAG_TDO   BDPROGSCRUDQP_EXT_CSF_1V8_FC_INNER   0.45888   2.647e-09 1.103e-12
AN33  UART2_RX   BDPROGSCARUDQP_SDMMC_STD_3V3SF_FC_OUTER  0.43813   2.597e-09 1.157e-12
AN35  UART0_TX   BDPROGSCARUDQP_SDMMC_STD_3V3SF_FC_OUTER  0.49304   2.940e-09 1.237e-12
AP2   DDR_DQS0_N   PDQS_PAD   0.59792   3.372e-09 1.374e-12
AP4   DDR_DQ05   PDDRIO_PAD_DATA   0.47751   2.741e-09 1.154e-12
AP6   DDR_DQ07   PDDRIO_PAD_DATA   0.4601   2.681e-09 1.104e-12
AP8   QSPI0A_SCLK   BDPROGSCARUDQP_SDMMC_STD_3V3SF_FC_OUTER  0.41178   2.509e-09 1.121e-12
AP10  QSPI0B_DATA0   BDPROGSCARUDQP_SDMMC_STD_3V3SF_FC_OUTER  0.4487   2.698e-09 1.184e-12
AP12  QSPI0B_DATA1   BDPROGSCARUDQP_SDMMC_STD_3V3SF_FC_INNER  0.43707   2.580e-09 1.111e-12
AP14  QSPI0B_DATA3   BDPROGSCARUDQP_SDMMC_STD_3V3SF_FC_INNER  0.41216   2.480e-09 1.115e-12
AP16  SPI1_SCK   BDPROGSCARUDQP_SDMMC_STD_3V3SF_FC_INNER  0.34639   2.142e-09 1.006e-12
AP18  SPI1_SDI   BDPROGSCARUDQP_SDMMC_STD_3V3SF_FC_INNER  0.35935   2.224e-09 1.010e-12
AP20  SNVS_TAMPER_OUT3   NC   0.34123   2.120e-09 9.768e-13
AP22  SNVS_TAMPER_OUT0   NC   0.31995   2.099e-09 9.352e-13
AP24  SNVS_TAMPER_OUT1   NC   0.46957   2.817e-09 1.245e-12
AP26  SCU_GPIO0_01   BDPROGSCRUDQP_EXT_CSF_1V8_FC_OUTER   0.39727   2.403e-09 1.042e-12
AP28  PMIC_I2C_SDA   BDPROGSCRUDQP_EXT_CSF_1V8_FC_OUTER   0.47082   2.689e-09 1.116e-12
AP30  PMIC_I2C_SCL   BDPROGSCRUDQP_EXT_CSF_1V8_FC_INNER   0.49096   2.810e-09 1.168e-12
AP32  JTAG_TMS   BDPROGSCRUDQP_EXT_CSF_1V8_FC_INNER   0.50879   2.969e-09 1.255e-12
AP34  UART2_TX   BDPROGSCARUDQP_SDMMC_STD_3V3SF_FC_INNER  0.50036   2.931e-09 1.264e-12
AR1   VSS_MAIN   GND   NA   NA   NA
AR3   DDR_DQ04   PDDRIO_PAD_DATA   0.47426   2.770e-09 1.184e-12
AR5   DDR_DQ06   PDDRIO_PAD_DATA   0.46504   2.722e-09 1.161e-12
AR7   QSPI0B_SCLK   BDPROGSCARUDQP_SDMMC_STD_3V3SF_FC_INNER  0.41374   2.587e-09 1.133e-12
AR9   QSPI0A_DQS   BDPROGSCARUDQP_SDMMC_STD_3V3SF_FC_INNER  0.41359   2.536e-09 1.067e-12
AR11  QSPI0A_DATA0   BDPROGSCARUDQP_SDMMC_STD_3V3SF_FC_INNER  0.39486   2.430e-09 1.018e-12
AR13  QSPI0B_DATA2   BDPROGSCARUDQP_SDMMC_STD_3V3SF_FC_OUTER  0.49663   2.948e-09 1.269e-12
AR15  SPI1_CS0   BDPROGSCARUDQP_SDMMC_STD_3V3SF_FC_OUTER  0.32415   2.055e-09 9.370e-13
AR17  SPI1_SDO   BDPROGSCARUDQP_SDMMC_STD_3V3SF_FC_OUTER  0.33473   2.087e-09 9.823e-13
AR19  PMIC_ON_REQ   NC   0.42859   2.630e-09 1.153e-12
AR21  ON_OFF_BUTTON   NC   0.41857   2.558e-09 1.125e-12
AR23  SCU_BOOT_MODE0   BDPROGSCRUDQP_EXT_CSF_1V8_FC_INNER   0.44731   2.708e-09 1.192e-12
AR25  SCU_BOOT_MODE1   BDPROGSCRUDQP_EXT_CSF_1V8_FC_OUTER   0.44895   2.744e-09 1.162e-12
AR27  SCU_GPIO0_00   BDPROGSCRUDQP_EXT_CSF_1V8_FC_INNER   0.46034   2.788e-09 1.164e-12
AR29  POR_B   BDPROGSCRUDQP_EXT_CSF_1V8_FC_INNER   0.47807   2.890e-09 1.194e-12
AR31  JTAG_TDI   BDPROGSCRUDQP_EXT_CSF_1V8_FC_OUTER   0.49918   2.931e-09 1.191e-12
AR33  JTAG_TCK   BDPROGSCRUDQP_EXT_CSF_1V8_FC_OUTER   0.51932   3.015e-09 1.250e-12
AR35  VSS_MAIN   GND   NA   NA   NA
[Pin Mapping]   pulldown_ref   pullup_ref
A1   VSS_MAIN   NC
A3   VSS_MAIN   VDD_DDR_VDDQ
A5   VSS_MAIN   VDD_DDR_VDDQ
A7   VSS_MAIN   VDD_DDR_VDDQ
A9   VSS_MAIN   VDD_PCIE_DIG_1P
A11   VSS_MAIN   VDD_PCIE_LDO_1P
A13   VSS_MAIN   VDD_PCIE_LDO_1P
A15   NC   NC
A17   VSS_MAIN   VDD_USB_3P3
A19   VSS_MAIN   VDD_USB_3P3
A21   VSS_MAIN   VDD_EMMC0_1P8_3
A23   VSS_MAIN   VDD_EMMC0_1P8_3
A25   VSS_MAIN   VDD_EMMC0_1P8_3
A27   VSS_MAIN   VDD_EMMC0_1P8_3
A29   VSS_MAIN   VDD_USDHC1_VSEL
A31   VSS_MAIN   VDD_ENET0_1P8_3
A33   VSS_MAIN   VDD_ENET0_1P8_3
A35   VSS_MAIN   NC
B2   VSS_MAIN   VDD_DDR_VDDQ
B4   VSS_MAIN   VDD_DDR_VDDQ
B6   VSS_MAIN   VDD_DDR_VDDQ
B8   VSS_MAIN   VDD_PCIE_DIG_1P
B10   VSS_MAIN   VDD_PCIE_LDO_1P
B12   VSS_MAIN   VDD_PCIE_LDO_1P
B14   NC   NC
B16   VSS_MAIN   VDD_USB_3P3
B18   VSS_MAIN   VDD_USB_3P3
B20   VSS_MAIN   VDD_EMMC0_1P8_3
B22   VSS_MAIN   VDD_EMMC0_1P8_3
B24   VSS_MAIN   VDD_EMMC0_1P8_3
B26   VSS_MAIN   VDD_EMMC0_1P8_3
B28   VSS_MAIN   VDD_USDHC1_VSEL
B30   VSS_MAIN   VDD_USDHC1_VSEL
B32   VSS_MAIN   VDD_ENET0_1P8_3
B34   VSS_MAIN   VDD_ENET0_1P8_3
C1   VSS_MAIN   NC
C3   VSS_MAIN   NC
C5   VSS_MAIN   VDD_DDR_VDDQ
C7   VSS_MAIN   NC
C9   VSS_MAIN   VDD_PCIE_DIG_1P
C11   VSS_MAIN   NC
C13   VSS_MAIN   NC
C15   VSS_MAIN   NC
C17   VSS_MAIN   NC
C19   NC   NC
C21   VSS_MAIN   VDD_EMMC0_1P8_3
C23   VSS_MAIN   VDD_EMMC0_1P8_3
C25   VSS_MAIN   VDD_EMMC0_1P8_3
C27   VSS_MAIN   VDD_EMMC0_1P8_3
C29   VSS_MAIN   VDD_USDHC1_VSEL
C31   VSS_MAIN   VDD_ENET0_1P8_3
C33   VSS_MAIN   VDD_ENET0_1P8_3
C35   VSS_MAIN   VDD_ENET0_VSELE
D2   VSS_MAIN   NC
D34   VSS_MAIN   VDD_ENET_MDIO_1
E1   VSS_MAIN   VDD_DDR_VDDQ
E3   VSS_MAIN   VDD_DDR_VDDQ
E5   VSS_MAIN   NC
E7   VSS_MAIN   NC
E9   VSS_MAIN   NC
E11   NC   VDD_PCIE_LDO_1P
E13   VSS_MAIN   NC
E15   NC   VDD_ANA0_1P8
E17   VSS_MAIN   NC
E19   VSS_MAIN   NC
E21   VSS_MAIN   NC
E23   VSS_MAIN   NC
E25   VSS_MAIN   NC
E27   VSS_MAIN   NC
E29   VSS_MAIN   NC
E31   VSS_MAIN   NC
E33   VSS_MAIN   VDD_ENET_MDIO_1
E35   VSS_MAIN   VDD_ENET_MDIO_1
F2   VSS_MAIN   VDD_DDR_VDDQ
F34   VSS_MAIN   VDD_ESAI_SPDIF_
G1   VSS_MAIN   VDD_DDR_VDDQ
G3   VSS_MAIN   NC
G5   VSS_MAIN   NC
G9   NC   NC
G11   NC   NC
G13   VSS_MAIN   VDD_USB_3P3
G15   NC   NC
G17   VSS_MAIN   VDD_USB_3P3
G19   VSS_MAIN   VDD_USB_3P3
G21   VSS_MAIN   VDD_USB_3P3
G23   VSS_MAIN   VDD_USB_3P3
G25   VSS_MAIN   VDD_USB_3P3
G27   VSS_MAIN   VDD_ENET0_VSELE
G29   VSS_MAIN   VDD_ENET0_VSELE
G31   VSS_MAIN   NC
G33   VSS_MAIN   VDD_ESAI_SPDIF_
G35   VSS_MAIN   VDD_ESAI_SPDIF_
H2   VSS_MAIN   VDD_DDR_VDDQ
H34   VSS_MAIN   VDD_ESAI_SPDIF_
J1   VSS_MAIN   VDD_DDR_VDDQ
J3   VSS_MAIN   VDD_DDR_VDDQ
J5   VSS_MAIN   NC
J7   VSS_MAIN   VDD_DDR_VDDQ
J9   VSS_MAIN   VDD_DDR_VDDQ
J11   VSS_MAIN   NC
J13   NC   VDD_PCIE_LDO_1P
J17   NC   VDD_USB_3P3
J19   NC   VDD_USB_3P3
J21   NC   VDD_USB_3P3
J23   NC   VDD_EMMC0_1P8_3
J25   NC   VDD_EMMC0_1P8_3
J27   NC   VDD_USDHC1_VSEL
J29   VSS_MAIN   VDD_ENET0_VSELE
J31   VSS_MAIN   NC
J33   VSS_MAIN   VDD_ESAI_SPDIF_
J35   VSS_MAIN   VDD_ESAI_SPDIF_
K2   VSS_MAIN   VDD_DDR_VDDQ
K34   VSS_MAIN   VDD_ESAI_SPDIF_
L1   VSS_MAIN   VDD_DDR_VDDQ
L3   VSS_MAIN   NC
L5   VSS_MAIN   NC
L7   VSS_MAIN   VDD_DDR_VDDQ
L9   NC   VDD_PCIE_DIG_1P
L11   VSS_MAIN   NC
L13   VSS_MAIN   NC
L15   VSS_MAIN   NC
L17   VSS_MAIN   NC
L19   VSS_MAIN   NC
L21   VSS_MAIN   NC
L23   VSS_MAIN   NC
L25   VSS_MAIN   NC
L27   NC   VDD_ENET0_VSELE
L29   VSS_MAIN   VDD_ENET0_VSELE
L31   VSS_MAIN   NC
L33   VSS_MAIN   VDD_ESAI_SPDIF_
L35   VSS_MAIN   VDD_ESAI_SPDIF_
M2   VSS_MAIN   VDD_DDR_VDDQ
M34   VSS_MAIN   VDD_ESAI_SPDIF_
N1   VSS_MAIN   VDD_DDR_VDDQ
N3   VSS_MAIN   VDD_DDR_VDDQ
N5   VSS_MAIN   NC
N7   NC   VDD_DDR_VDDQ
N9   NC   VDD_DDR_VDDQ
N11   VSS_MAIN   NC
N13   NC   VDD_DDR_VDDQ
N15   NC   VDD_ENET0_1P8_3
N17   NC   VDD_ENET0_1P8_3
N19   NC   VDD_ENET0_1P8_3
N21   NC   VDD_ENET0_1P8_3
N23   NC   VDD_ENET0_1P8_3
N25   VSS_MAIN   NC
N27   NC   VDD_ENET0_1P8_3
N29   VSS_MAIN   VDD_ENET0_VSELE
N31   VSS_MAIN   NC
N33   VSS_MAIN   VDD_ESAI_SPDIF_
N35   VSS_MAIN   VDD_ESAI_SPDIF_
P2   VSS_MAIN   VDD_DDR_VDDQ
P34   VSS_MAIN   VDD_SPI_MCLK_UA
R1   VSS_MAIN   VDD_DDR_VDDQ
R3   VSS_MAIN   NC
R5   VSS_MAIN   NC
R7   NC   VDD_DDR_VDDQ
R9   NC   VDD_DDR_VDDQ
R11   VSS_MAIN   NC
R13   NC   VDD_DDR_VDDQ
R15   NC   VDD_ENET0_1P8_3
R17   NC   VDD_ENET0_1P8_3
R19   VSS_MAIN   NC
R21   VSS_MAIN   NC
R23   NC   VDD_ENET0_1P8_3
R25   VSS_MAIN   NC
R27   NC   VDD_ENET_MDIO_1
R29   VSS_MAIN   VDD_ESAI_SPDIF_
R31   VSS_MAIN   NC
R33   VSS_MAIN   VDD_SPI_MCLK_UA
R35   VSS_MAIN   VDD_SPI_MCLK_UA
T2   VSS_MAIN   VDD_DDR_VDDQ
T34   VSS_MAIN   VDD_SPI_MCLK_UA
U1   VSS_MAIN   VDD_DDR_VDDQ
U3   VSS_MAIN   VDD_DDR_VDDQ
U5   VSS_MAIN   NC
U7   NC   VDD_DDR_VDDQ
U9   NC   VDD_DDR_VDDQ
U11   VSS_MAIN   NC
U13   NC   VDD_DDR_VDDQ
U15   VSS_MAIN   NC
U17   VSS_MAIN   NC
U19   NC   VDD_DDR_VDDQ
U21   VSS_MAIN   NC
U23   NC   VDD_ENET0_1P8_3
U25   VSS_MAIN   NC
U27   NC   VDD_ESAI_SPDIF_
U29   VSS_MAIN   VDD_SPI_MCLK_UA
U31   VSS_MAIN   NC
U33   VSS_MAIN   VDD_SPI_MCLK_UA
U35   VSS_MAIN   VDD_SPI_MCLK_UA
V2   VSS_MAIN   VDD_DDR_VDDQ
V34   VSS_MAIN   VDD_SPI_MCLK_UA
W1   VSS_MAIN   VDD_DDR_VDDQ
W3   VSS_MAIN   NC
W5   VSS_MAIN   NC
W7   NC   VDD_DDR_VDDQ
W9   NC   VDD_DDR_VDDQ
W11   VSS_MAIN   NC
W13   NC   VDD_DDR_VDDQ
W15   NC   VDD_DDR_VDDQ
W17   NC   VDD_DDR_VDDQ
W19   NC   VDD_DDR_VDDQ
W21   VSS_MAIN   NC
W23   NC   VDD_ENET0_1P8_3
W25   VSS_MAIN   NC
W27   NC   VDD_SPI_MCLK_UA
W29   VSS_MAIN   VDD_SPI_MCLK_UA
W31   VSS_MAIN   NC
W33   VSS_MAIN   VDD_SPI_MCLK_UA
W35   VSS_MAIN   VDD_SPI_MCLK_UA
Y2   VSS_MAIN   VDD_DDR_VDDQ
Y34   VSS_MAIN   VDD_SPI_SAI_1P8
AA1   VSS_MAIN   VDD_DDR_VDDQ
AA3   VSS_MAIN   VDD_DDR_VDDQ
AA5   VSS_MAIN   NC
AA7   NC   VDD_DDR_VDDQ
AA9   NC   VDD_DDR_VDDQ
AA11   VSS_MAIN   NC
AA13   NC   VDD_DDR_VDDQ
AA15   VSS_MAIN   NC
AA17   VSS_MAIN   NC
AA19   VSS_MAIN   NC
AA21   VSS_MAIN   NC
AA23   NC   VDD_ENET0_1P8_3
AA25   VSS_MAIN   NC
AA27   NC   VDD_SPI_SAI_1P8
AA29   VSS_MAIN   VDD_SPI_MCLK_UA
AA31   VSS_MAIN   NC
AA33   VSS_MAIN   VDD_SPI_SAI_1P8
AA35   VSS_MAIN   VDD_SPI_SAI_1P8
AB2   VSS_MAIN   VDD_DDR_VDDQ
AB34   VSS_MAIN   VDD_SPI_SAI_1P8
AC1   VSS_MAIN   VDD_DDR_VDDQ
AC3   VSS_MAIN   NC
AC5   VSS_MAIN   NC
AC7   NC   NC
AC9   NC   VDD_DDR_VDDQ
AC11   VSS_MAIN   NC
AC13   NC   VDD_DDR_VDDQ
AC15   NC   VDD_DDR_VDDQ
AC17   NC   VDD_ENET0_1P8_3
AC19   NC   VDD_ENET0_1P8_3
AC21   NC   VDD_ENET0_1P8_3
AC23   NC   VDD_ENET0_1P8_3
AC25   VSS_MAIN   NC
AC27   NC   VDD_ADC_DIG_1P8
AC29   NC   VDD_ADC_DIG_1P8
AC31   VSS_MAIN   NC
AC33   VSS_MAIN   VDD_ADC_DIG_1P8
AC35   VSS_MAIN   VDD_SPI_SAI_1P8
AD2   VSS_MAIN   VDD_DDR_VDDQ
AD34   VSS_MAIN   VDD_ADC_DIG_1P8
AE1   VSS_MAIN   VDD_DDR_VDDQ
AE3   VSS_MAIN   VDD_DDR_VDDQ
AE5   VSS_MAIN   NC
AE7   NC   VDD_DDR_VDDQ
AE9   NC   VDD_DDR_VDDQ
AE11   VSS_MAIN   NC
AE13   VSS_MAIN   NC
AE15   VSS_MAIN   NC
AE17   VSS_MAIN   NC
AE19   VSS_MAIN   NC
AE21   VSS_MAIN   NC
AE23   VSS_MAIN   NC
AE25   VSS_MAIN   NC
AE27   NC   VDD_ADC_DIG_1P8
AE29   VSS_MAIN   NC
AE31   VSS_MAIN   NC
AE33   VSS_MAIN   VDD_ADC_DIG_1P8
AE35   VSS_MAIN   VDD_ADC_DIG_1P8
AF2   VSS_MAIN   VDD_DDR_VDDQ
AF34   VSS_MAIN   VDD_ADC_DIG_1P8
AG1   VSS_MAIN   VDD_DDR_VDDQ
AG3   VSS_MAIN   NC
AG5   VSS_MAIN   NC
AG7   VSS_MAIN   VDD_DDR_VDDQ
AG9   VSS_MAIN   VDD_DDR_VDDQ
AG11   NC   VDD_QSPI0B_1P8_
AG13   NC   VDD_QSPI0A_1P8_
AG15   NC   VDD_CSI_1P8_3P3
AG17   NC   VDD_TMPR_CSI_1P
AG19   NC   VDD_SNVS_LDO_1P
AG21   NC   NC
AG23   NC   NC
AG25   NC   NC
AG27   NC   VDD_CAN_UART_1P
AG29   VSS_MAIN   VDD_ANA1_1P8
AG31   VSS_MAIN   NC
AG33   VSS_MAIN   NC
AG35   VSS_MAIN   VDD_ADC_DIG_1P8
AH2   VSS_MAIN   VDD_DDR_VDDQ
AH34   VSS_MAIN   VDD_CAN_UART_1P
AJ1   VSS_MAIN   VDD_DDR_VDDQ
AJ3   VSS_MAIN   VDD_DDR_VDDQ
AJ5   VSS_MAIN   NC
AJ7   NC   NC
AJ9   NC   NC
AJ11   VSS_MAIN   VDD_QSPI0B_1P8_
AJ13   NC   NC
AJ15   NC   NC
AJ17   NC   NC
AJ19   NC   NC
AJ21   NC   NC
AJ23   NC   NC
AJ25   NC   NC
AJ27   NC   VDD_ANA1_1P8
AJ29   VSS_MAIN   VDD_ANA1_1P8
AJ31   VSS_MAIN   NC
AJ33   VSS_MAIN   VDD_CAN_UART_1P
AJ35   VSS_MAIN   VDD_CAN_UART_1P
AK2   VSS_MAIN   VDD_DDR_VDDQ
AK34   VSS_MAIN   VDD_CAN_UART_1P
AL1   VSS_MAIN   VDD_DDR_VDDQ
AL3   VSS_MAIN   NC
AL5   VSS_MAIN   NC
AL7   VSS_MAIN   NC
AL9   VSS_MAIN   NC
AL11   VSS_MAIN   NC
AL13   VSS_MAIN   NC
AL15   VSS_MAIN   NC
AL17   VSS_MAIN   NC
AL19   VSS_MAIN   NC
AL21   VSS_MAIN   NC
AL23   VSS_MAIN   NC
AL25   VSS_MAIN   NC
AL27   VSS_MAIN   NC
AL29   VSS_MAIN   NC
AL31   VSS_MAIN   NC
AL33   VSS_MAIN   VDD_CAN_UART_1P
AL35   VSS_MAIN   VDD_CAN_UART_1P
AM2   VSS_MAIN   VDD_DDR_VDDQ
AM34   VSS_MAIN   VDD_CAN_UART_1P
AN1   VSS_MAIN   VDD_DDR_VDDQ
AN3   VSS_MAIN   VDD_DDR_VDDQ
AN5   VSS_MAIN   NC
AN7   VSS_MAIN   VDD_QSPI0A_1P8_
AN9   VSS_MAIN   VDD_QSPI0A_1P8_
AN11   VSS_MAIN   VDD_QSPI0A_1P8_
AN13   VSS_MAIN   VDD_QSPI0A_1P8_
AN15   VSS_MAIN   VDD_QSPI0B_1P8_
AN17   NC   NC
AN19   NC   NC
AN21   NC   NC
AN23   NC   NC
AN25   VSS_MAIN   VDD_ANA1_1P8
AN27   VSS_MAIN   VDD_ANA1_1P8
AN29   VSS_MAIN   VDD_ANA1_1P8
AN31   VSS_MAIN   VDD_ANA1_1P8
AN33   VSS_MAIN   VDD_CAN_UART_1P
AN35   VSS_MAIN   VDD_CAN_UART_1P
AP2   VSS_MAIN   VDD_DDR_VDDQ
AP4   VSS_MAIN   VDD_DDR_VDDQ
AP6   VSS_MAIN   VDD_DDR_VDDQ
AP8   VSS_MAIN   VDD_QSPI0A_1P8_
AP10   VSS_MAIN   VDD_QSPI0B_1P8_
AP12   VSS_MAIN   VDD_QSPI0B_1P8_
AP14   VSS_MAIN   VDD_QSPI0B_1P8_
AP16   VSS_MAIN   VDD_CSI_1P8_3P3
AP18   VSS_MAIN   VDD_CSI_1P8_3P3
AP20   NC   NC
AP22   NC   NC
AP24   NC   NC
AP26   VSS_MAIN   VDD_ANA1_1P8
AP28   VSS_MAIN   VDD_ANA1_1P8
AP30   VSS_MAIN   VDD_ANA1_1P8
AP32   VSS_MAIN   VDD_ANA1_1P8
AP34   VSS_MAIN   VDD_CAN_UART_1P
AR1   VSS_MAIN   NC
AR3   VSS_MAIN   VDD_DDR_VDDQ
AR5   VSS_MAIN   VDD_DDR_VDDQ
AR7   VSS_MAIN   VDD_QSPI0B_1P8_
AR9   VSS_MAIN   VDD_QSPI0A_1P8_
AR11   VSS_MAIN   VDD_QSPI0A_1P8_
AR13   VSS_MAIN   VDD_QSPI0B_1P8_
AR15   VSS_MAIN   VDD_CSI_1P8_3P3
AR17   VSS_MAIN   VDD_CSI_1P8_3P3
AR19   NC   NC
AR21   NC   NC
AR23   VSS_MAIN   VDD_ANA1_1P8
AR25   VSS_MAIN   VDD_ANA1_1P8
AR27   VSS_MAIN   VDD_ANA1_1P8
AR29   VSS_MAIN   VDD_ANA1_1P8
AR31   VSS_MAIN   VDD_ANA1_1P8
AR33   VSS_MAIN   VDD_ANA1_1P8
AR35   VSS_MAIN   NC
[Diff Pin]  inv_pin  vdiff  tdelay_typ tdelay_min tdelay_max
A11   B10   NA   NA   NA   NA
A13   B12   NA   NA   NA   NA
A17   B16   NA   NA   NA   NA
B18   A19   NA   NA   NA   NA
L1   K2   NA   NA   NA   NA
AE3   AD2   NA   NA   NA   NA
AN1   AP2   NA   NA   NA   NA
|*   Model Selector   *
[Model Selector] ABI_SERDES
abi_out   ABI Serdes output
abi_in   ABI Serdes input
[Model Selector] BDPROGSCARUDQP_SDMMC_STD_3V3SF_FC_INNER
BDPROGSCARUDQP_SDMMC_3V3SF_00_SD   PSW=0 PDRV=0 MODE=1V8 SD
BDPROGSCARUDQP_SDMMC_3V3SF_01_SD   PSW=0 PDRV=1 MODE=1V8 SD
BDPROGSCARUDQP_SDMMC_3V3SF_00_MMC   PSW=0 PDRV=0 MODE=1V8 MMC
BDPROGSCARUDQP_SDMMC_3V3SF_01_MMC   PSW=0 PDRV=1 MODE=1V8 MMC
BDPROGSCARUDQP_SDMMC_3V3SF_10   PSW=1 PDRV=0 MODE=3V3 SD & 3V3 MMC
BDPROGSCARUDQP_SDMMC_3V3SF_11   PSW=1 PDRV=1 MODE=3V3 SD & 3V3 MMC
BDPROGSCARUDQP_SDMMC_3V3SF_11_2v7   PSW=1 PDRV=1 MODE=2V7 SD & 2V7 MMC
BDPROGSCARUDQP_SDMMC_3V3SF_10_2v7   PSW=1 PDRV=0 MODE=2V7 SD & 2V7 MMC
[Model Selector] BDPROGSCARUDQP_SDMMC_STD_3V3SF_FC_OUTER
BDPROGSCARUDQP_SDMMC_3V3SF_00_SD   PSW=0 PDRV=0 MODE=1V8 SD
BDPROGSCARUDQP_SDMMC_3V3SF_01_SD   PSW=0 PDRV=1 MODE=1V8 SD
BDPROGSCARUDQP_SDMMC_3V3SF_00_MMC   PSW=0 PDRV=0 MODE=1V8 MMC
BDPROGSCARUDQP_SDMMC_3V3SF_01_MMC   PSW=0 PDRV=1 MODE=1V8 MMC
BDPROGSCARUDQP_SDMMC_3V3SF_10   PSW=1 PDRV=0 MODE=3V3 SD & 3V3 MMC
BDPROGSCARUDQP_SDMMC_3V3SF_11   PSW=1 PDRV=1 MODE=3V3 SD & 3V3 MMC
BDPROGSCARUDQP_SDMMC_3V3SF_11_2v7   PSW=1 PDRV=1 MODE=2V7 SD & 2V7 MMC
BDPROGSCARUDQP_SDMMC_3V3SF_10_2v7   PSW=1 PDRV=0 MODE=2V7 SD & 2V7 MMC
[Model Selector] BDPROGSCRUDQP_EXT_CSF_1V8_FC_INNER
BDPROG_1V2_000   [1V2 DRIVE2=0  DRIVE1=0  DRIVE0=0]
BDPROG_1V2_001   [1V2 DRIVE2=0  DRIVE1=0  DRIVE0=1]
BDPROG_1V2_010   [1V2 DRIVE2=0  DRIVE1=1  DRIVE0=0]
BDPROG_1V2_011   [1V2 DRIVE2=0  DRIVE1=1  DRIVE0=1]
BDPROG_1V2_100   [1V2 DRIVE2=1  DRIVE1=0  DRIVE0=0]
BDPROG_1V2_101   [1V2 DRIVE2=1  DRIVE1=0  DRIVE0=1]
BDPROG_1V2_110   [1V2 DRIVE2=1  DRIVE1=1  DRIVE0=0]
BDPROG_1V2_111   [1V2 DRIVE2=1  DRIVE1=1  DRIVE0=1]
BDPROG_1V8_000   [1V8 DRIVE2=0  DRIVE1=0  DRIVE0=0]
BDPROG_1V8_001   [1V8 DRIVE2=0  DRIVE1=0  DRIVE0=1]
BDPROG_1V8_010   [1V8 DRIVE2=0  DRIVE1=1  DRIVE0=0]
BDPROG_1V8_011   [1V8 DRIVE2=0  DRIVE1=1  DRIVE0=1]
BDPROG_1V8_100   [1V8 DRIVE2=1  DRIVE1=0  DRIVE0=0]
BDPROG_1V8_101   [1V8 DRIVE2=1  DRIVE1=0  DRIVE0=1]
BDPROG_1V8_110   [1V8 DRIVE2=1  DRIVE1=1  DRIVE0=0]
BDPROG_1V8_111   [1V8 DRIVE2=1  DRIVE1=1  DRIVE0=1]
[Model Selector] BDPROGSCRUDQP_EXT_CSF_1V8_FC_OUTER
BDPROG_1V2_000   [1V2 DRIVE2=0  DRIVE1=0  DRIVE0=0]
BDPROG_1V2_001   [1V2 DRIVE2=0  DRIVE1=0  DRIVE0=1]
BDPROG_1V2_010   [1V2 DRIVE2=0  DRIVE1=1  DRIVE0=0]
BDPROG_1V2_011   [1V2 DRIVE2=0  DRIVE1=1  DRIVE0=1]
BDPROG_1V2_100   [1V2 DRIVE2=1  DRIVE1=0  DRIVE0=0]
BDPROG_1V2_101   [1V2 DRIVE2=1  DRIVE1=0  DRIVE0=1]
BDPROG_1V2_110   [1V2 DRIVE2=1  DRIVE1=1  DRIVE0=0]
BDPROG_1V2_111   [1V2 DRIVE2=1  DRIVE1=1  DRIVE0=1]
BDPROG_1V8_000   [1V8 DRIVE2=0  DRIVE1=0  DRIVE0=0]
BDPROG_1V8_001   [1V8 DRIVE2=0  DRIVE1=0  DRIVE0=1]
BDPROG_1V8_010   [1V8 DRIVE2=0  DRIVE1=1  DRIVE0=0]
BDPROG_1V8_011   [1V8 DRIVE2=0  DRIVE1=1  DRIVE0=1]
BDPROG_1V8_100   [1V8 DRIVE2=1  DRIVE1=0  DRIVE0=0]
BDPROG_1V8_101   [1V8 DRIVE2=1  DRIVE1=0  DRIVE0=1]
BDPROG_1V8_110   [1V8 DRIVE2=1  DRIVE1=1  DRIVE0=0]
BDPROG_1V8_111   [1V8 DRIVE2=1  DRIVE1=1  DRIVE0=1]
[Model Selector] PCKE_PAD
DWC_D5MC3L_34   DDR3L DWC_D5M_PCKE cell  Z0=34-Ohm
DWC_D5MC3L_40   DDR3L DWC_D5M_PCKE cell  Z0=40-Ohm
DWC_D5MC3L_48   DDR3L DWC_D5M_PCKE cell  Z0=48-Ohm
DWC_D5MC3L_ODT40   DDR3L DWC_D5M_PCKE cell 40-Ohm ODT Receiver
DWC_D5MC3L_ODT60   DDR3L DWC_D5M_PCKE cell 60-Ohm ODT Receiver
DWC_D5MC3L_ODTOFF   DDR3L DWC_D5M_PCKE cell ODT off Receiver
DWC_D5MC3_34   DDR3 DWC_D5M_PCKE cell  Z0=34-Ohm
DWC_D5MC3_40   DDR3 DWC_D5M_PCKE cell  Z0=40-Ohm
DWC_D5MC3_48   DDR3 DWC_D5M_PCKE cell  Z0=48-Ohm
DWC_D5MC3_ODT40   DDR3 DWC_D5M_PCKE cell 40-Ohm ODT Receiver
DWC_D5MC3_ODT60   DDR3 DWC_D5M_PCKE cell 60-Ohm ODT Receiver
DWC_D5MC3_ODTOFF   DDR3 DWC_D5M_PCKE cell ODT off Receiver
DWC_D5MC4_34   DDR4 DWC_D5M_PCKE cell Supply-terminated  Z0=34-Ohm Driver SR=00
DWC_D5MC4_34M   DDR4 DWC_D5M_PCKE cell Mid-rail terminated  Z0=34-Ohm Driver SR=00
DWC_D5MC4_34M_TXM   DDR4 DWC_D5M_PCKE cell Mid-rail terminated  Z0=34-Ohm Driver SR=11 Pre-emphasis ON
DWC_D5MC4_34ODT40   DDR4 DWC_D5M_PCKE Supply-terminated cell 40-Ohm ODT Receiver
DWC_D5MC4_34ODTOFF   DDR4 DWC_D5M_PCKE Supply-terminated cell ODT OFF Receiver
DWC_D5MC4_34_TXM   DDR4 DWC_D5M_PCKE cell Supply-terminated  Z0=34-Ohm Driver SR=11 Pre-emphasis ON
DWC_D5MC4_48   DDR4 DWC_D5M_PCKE cell Supply-terminated  Z0=48-Ohm Driver SR=00
DWC_D5MC4_48M   DDR4 DWC_D5M_PCKE cell Mid-rail terminated  Z0=48-Ohm Driver SR=00
DWC_D5MC4_48M_TXM   DDR4 DWC_D5M_PCKE cell Mid-rail terminated  Z0=48-Ohm Driver SR=11 Pre-emphasis ON
DWC_D5MC4_48ODT60   DDR4 DWC_D5M_PCKE Supply-terminated cell 60-Ohm ODT Receiver
DWC_D5MC4_48_TXM   DDR4 DWC_D5M_PCKE cell Supply-terminated  Z0=48-Ohm Driver SR=11 Pre-emphasis ON
DWC_D5MCL2_34   LPDDR2 DWC_D5M_PCKE cell  Z0=34-Ohm
DWC_D5MCL2_48   LPDDR2 DWC_D5M_PCKE cell  Z0=48-Ohm
DWC_D5MCL2_ODTOFF   LPDDR2 DWC_D5M_PCKE cell ODT off Receiver
DWC_D5MCL3_34   LPDDR3 DWC_D5M_PCKE Supply-reminated cell  Z0=34-Ohm
DWC_D5MCL3_34M   LPDDR3 DWC_D5M_PCKE Mid-rail terminated cell  Z0=34-Ohm
DWC_D5MCL3_34ODT120   LPDDR3 DWC_D5M_PCKE cell ODT 120 Ohms Receiver
DWC_D5MCL3_34ODT240   LPDDR3 DWC_D5M_PCKE cell ODT 240 Ohms Receiver
DWC_D5MCL3_34ODT60   LPDDR3 DWC_D5M_PCKE Supply-terminated cell ODT 60 Ohms Receiver
DWC_D5MCL3_34ODTOFF   LPDDR3 DWC_D5M_PCKE cell ODT off Receiver
DWC_D5MCL3_40   LPDDR3 DWC_D5M_PCKE Supply-terminated cell  Z0=40-Ohm
DWC_D5MCL3_48   LPDDR3 DWC_D5M_PCKE Supply-terminated cell  Z0=48-Ohm
DWC_D5MCL3_48M   LPDDR3 DWC_D5M_PCKE Mid-rail terminated cell  Z0=48-Ohm
DWC_D5MCL3_ODT120M   LPDDR3 DWC_D5M_PCKE cell ODT 120 Ohms Receiver
DWC_D5MCL3_ODT240M   LPDDR3 DWC_D5M_PCKE cell ODT 240 Ohms Receiver
DWC_D5MCL4_40   LPDDR4 DWC_D5M_PCKE cell  Z0=40-Ohm Driver SR=00
DWC_D5MCL4_40_TXM   LPDDR4 DWC_D5M_PCKE cell  Z0=40-Ohm Driver SR=11 Pre-emphasis ON
DWC_D5MCL4_48   LPDDR4 DWC_D5M_PCKE cell  Z0=48-Ohm Driver SR=00
DWC_D5MCL4_48_TXM   LPDDR4 DWC_D5M_PCKE cell  Z0=48-Ohm Driver SR=11 Pre-emphasis ON
DWC_D5MCL4_60   LPDDR4 DWC_D5M_PCKE cell  Z0=60-Ohm Driver SR=00
DWC_D5MCL4_60_TXM   LPDDR4 DWC_D5M_PCKE cell  Z0=60-Ohm Driver SR=11 Pre-emphasis ON
DWC_D5MCL4_80   LPDDR4 DWC_D5M_PCKE cell  Z0=80-Ohm Driver SR=00
DWC_D5MCL4_80_TXM   LPDDR4 DWC_D5M_PCKE cell  Z0=80-Ohm Driver SR=11 Pre-emphasis ON
DWC_D5MCL4_ODT40   LPDDR4 DWC_D5M_PCKE cell 40-Ohm ODT Receiver
DWC_D5MCL4_ODT48   LPDDR4 DWC_D5M_PCKE cell 48-Ohm ODT Receiver
DWC_D5MCL4_ODT60   LPDDR4 DWC_D5M_PCKE cell 60-Ohm ODT Receiver
DWC_D5MCL4_ODT80   LPDDR4 DWC_D5M_PCKE cell 80-Ohm ODT Receiver
DWC_D5MCL4_ODTOFF   LPDDR4 DWC_D5M_PCKE cell  ODT off Receiver
[Model Selector] PCK_PAD
DWC_D5MCK3L_34   DDR3L DWC_D5M_PCK cell  Z0=34-Ohm
DWC_D5MCK3L_40   DDR3L DWC_D5M_PCK cell  Z0=40-Ohm
DWC_D5MCK3L_48   DDR3L DWC_D5M_PCK cell  Z0=48-Ohm
DWC_D5MCK3L_ODT40   DDR3L DWC_D5M_PCK cell 40-Ohm ODT Receiver
DWC_D5MCK3L_ODT60   DDR3L DWC_D5M_PCK cell 60-Ohm ODT Receiver
DWC_D5MCK3L_ODTOFF   DDR3L DWC_D5M_PCK cell ODT off Receiver
DWC_D5MCK3_34   DDR3 DWC_D5M_PCK cell  Z0=34-Ohm
DWC_D5MCK3_40   DDR3 DWC_D5M_PCK cell  Z0=40-Ohm
DWC_D5MCK3_48   DDR3 DWC_D5M_PCK cell  Z0=48-Ohm
DWC_D5MCK3_ODT40   DDR3 DWC_D5M_PCK cell 40-Ohm ODT Receiver
DWC_D5MCK3_ODT60   DDR3 DWC_D5M_PCK cell 60-Ohm ODT Receiver
DWC_D5MCK3_ODTOFF   DDR3 DWC_D5M_PCK cell ODT off Receiver
DWC_D5MCK4_34   DDR4 DWC_D5M_PCK cell Supply-terminated  Z0=34-Ohm Driver SR=00
DWC_D5MCK4_34M   DDR4 DWC_D5M_PCK cell Mid-rail terminated  Z0=34-Ohm Driver SR=00
DWC_D5MCK4_34M_TXM   DDR4 DWC_D5M_PCK cell Mid-rail terminated  Z0=34-Ohm Driver SR=11 Pre-emphasis ON
DWC_D5MCK4_34ODT40   DDR4 DWC_D5M_PCK Supply-terminated cell 40-Ohm ODT Receiver
DWC_D5MCK4_34ODTOFF   DDR4 DWC_D5M_PCK Supply-terminated cell ODT OFF Receiver
DWC_D5MCK4_34_TXM   DDR4 DWC_D5M_PCK cell Supply-terminated  Z0=34-Ohm Driver SR=11 Pre-emphasis ON
DWC_D5MCK4_48   DDR4 DWC_D5M_PCK cell Supply-terminated  Z0=48-Ohm Driver SR=00
DWC_D5MCK4_48M   DDR4 DWC_D5M_PCK cell Mid-rail terminated  Z0=48-Ohm Driver SR=00
DWC_D5MCK4_48M_TXM   DDR4 DWC_D5M_PCK cell Mid-rail terminated  Z0=48-Ohm Driver SR=11 Pre-emphasis ON
DWC_D5MCK4_48ODT60   DDR4 DWC_D5M_PCK Supply-terminated cell 60-Ohm ODT Receiver
DWC_D5MCK4_48_TXM   DDR4 DWC_D5M_PCK cell Supply-terminated  Z0=48-Ohm Driver SR=11 Pre-emphasis ON
DWC_D5MCKL2_34   LPDDR2 DWC_D5M_PCK cell  Z0=34-Ohm
DWC_D5MCKL2_48   LPDDR2 DWC_D5M_PCK cell  Z0=48-Ohm
DWC_D5MCKL2_ODTOFF   LPDDR2 DWC_D5M_PCK cell ODT off Receiver
DWC_D5MCKL3_34   LPDDR3 DWC_D5M_PCK Supply-reminated cell  Z0=34-Ohm
DWC_D5MCKL3_34M   LPDDR3 DWC_D5M_PCK Mid-rail terminated cell  Z0=34-Ohm
DWC_D5MCKL3_34ODT120   LPDDR3 DWC_D5M_PCK cell ODT 120 Ohms Receiver
DWC_D5MCKL3_34ODT240   LPDDR3 DWC_D5M_PCK cell ODT 240 Ohms Receiver
DWC_D5MCKL3_34ODT60   LPDDR3 DWC_D5M_PCK Supply-terminated cell ODT 60 Ohms Receiver
DWC_D5MCKL3_34ODTOFF   LPDDR3 DWC_D5M_PCK cell ODT off Receiver
DWC_D5MCKL3_40   LPDDR3 DWC_D5M_PCK Supply-terminated cell  Z0=40-Ohm
DWC_D5MCKL3_48   LPDDR3 DWC_D5M_PCK Supply-terminated cell  Z0=48-Ohm
DWC_D5MCKL3_48M   LPDDR3 DWC_D5M_PCK Mid-rail terminated cell  Z0=48-Ohm
DWC_D5MCKL3_ODT120M   LPDDR3 DWC_D5M_PCK cell ODT 120 Ohms Receiver
DWC_D5MCKL3_ODT240M   LPDDR3 DWC_D5M_PCK cell ODT 240 Ohms Receiver
DWC_D5MCKL4_40   LPDDR4 DWC_D5M_PCK cell  Z0=40-Ohm Driver SR=00
DWC_D5MCKL4_40_TXM   LPDDR4 DWC_D5M_PCK cell  Z0=40-Ohm Driver SR=11 Pre-emphasis ON
DWC_D5MCKL4_48   LPDDR4 DWC_D5M_PCK cell  Z0=48-Ohm Driver SR=00
DWC_D5MCKL4_48_TXM   LPDDR4 DWC_D5M_PCK cell  Z0=48-Ohm Driver SR=11 Pre-emphasis ON
DWC_D5MCKL4_60   LPDDR4 DWC_D5M_PCK cell  Z0=60-Ohm Driver SR=00
DWC_D5MCKL4_60_TXM   LPDDR4 DWC_D5M_PCK cell  Z0=60-Ohm Driver SR=11 Pre-emphasis ON
DWC_D5MCKL4_80   LPDDR4 DWC_D5M_PCK cell  Z0=80-Ohm Driver SR=00
DWC_D5MCKL4_80_TXM   LPDDR4 DWC_D5M_PCK cell  Z0=80-Ohm Driver SR=11 Pre-emphasis ON
DWC_D5MCKL4_ODT40   LPDDR4 DWC_D5M_PCK cell 40-Ohm ODT Receiver
DWC_D5MCKL4_ODT48   LPDDR4 DWC_D5M_PCK cell 48-Ohm ODT Receiver
DWC_D5MCKL4_ODT60   LPDDR4 DWC_D5M_PCK cell 60-Ohm ODT Receiver
DWC_D5MCKL4_ODT80   LPDDR4 DWC_D5M_PCK cell 80-Ohm ODT Receiver
DWC_D5MCKL4_ODTOFF   LPDDR4 DWC_D5M_PCK cell  ODT off Receiver
[Model Selector] PDDRIO_PAD_COMMAND
DWC_D5MP3L_34   DDR3L DWC_D5M_PDDRIO cell  Z0=34-Ohm
DWC_D5MP3L_40   DDR3L DWC_D5M_PDDRIO cell  Z0=40-Ohm
DWC_D5MP3L_48   DDR3L DWC_D5M_PDDRIO cell  Z0=48-Ohm
DWC_D5MP3L_60   DDR3L DWC_D5M_PDDRIO cell  Z0=60-Ohm Driver SR=00
DWC_D5MP3L_60_TXM   DDR3L DWC_D5M_PDDRIO cell  Z0=60-Ohm Driver SR=11 Pre-emphasis ON
DWC_D5MP3L_ODT40   DDR3L DWC_D5M_PDDRIO cell 40-Ohm ODT Receiver
DWC_D5MP3L_ODT60   DDR3L DWC_D5M_PDDRIO cell 60-Ohm ODT Receiver
DWC_D5MP3L_ODTOFF   DDR3L DWC_D5M_PDDRIO cell ODT off Receiver
DWC_D5MP3_34   DDR3 DWC_D5M_PDDRIO cell  Z0=34-Ohm
DWC_D5MP3_40   DDR3 DWC_D5M_PDDRIO cell  Z0=40-Ohm
DWC_D5MP3_48   DDR3 DWC_D5M_PDDRIO cell  Z0=48-Ohm
DWC_D5MP3_ODT40   DDR3 DWC_D5M_PDDRIO cell 40-Ohm ODT Receiver
DWC_D5MP3_ODT60   DDR3 DWC_D5M_PDDRIO cell 60-Ohm ODT Receiver
DWC_D5MP3_ODTOFF   DDR3 DWC_D5M_PDDRIO cell ODT off Receiver
DWC_D5MP4_34   DDR4 DWC_D5M_PDDRIO cell Supply-terminated  Z0=34-Ohm Driver SR=00
DWC_D5MP4_34M   DDR4 DWC_D5M_PDDRIO cell Mid-rail terminated  Z0=34-Ohm Driver SR=00
DWC_D5MP4_34M_TXM   DDR4 DWC_D5M_PDDRIO cell Mid-rail terminated  Z0=34-Ohm Driver SR=11 Pre-emphasis ON
DWC_D5MP4_34ODT40   DDR4 DWC_D5M_PDDRIO Supply-terminated cell 40-Ohm ODT Receiver
DWC_D5MP4_34ODTOFF   DDR4 DWC_D5M_PDDRIO Supply-terminated cell ODT OFF Receiver
DWC_D5MP4_34_TXM   DDR4 DWC_D5M_PDDRIO cell Supply-terminated  Z0=34-Ohm Driver SR=11 Pre-emphasis ON
DWC_D5MP4_48   DDR4 DWC_D5M_PDDRIO cell Supply-terminated  Z0=48-Ohm Driver SR=00
DWC_D5MP4_48M   DDR4 DWC_D5M_PDDRIO cell Mid-rail terminated  Z0=48-Ohm Driver SR=00
DWC_D5MP4_48M_TXM   DDR4 DWC_D5M_PDDRIO cell Mid-rail terminated  Z0=48-Ohm Driver SR=11 Pre-emphasis ON
DWC_D5MP4_48ODT60   DDR4 DWC_D5M_PDDRIO Supply-terminated cell 60-Ohm ODT Receiver
DWC_D5MP4_48_TXM   DDR4 DWC_D5M_PDDRIO cell Supply-terminated  Z0=48-Ohm Driver SR=11 Pre-emphasis ON
DWC_D5MPL2_34   LPDDR2 DWC_D5M_PDDRIO cell  Z0=34-Ohm
DWC_D5MPL2_48   LPDDR2 DWC_D5M_PDDRIO cell  Z0=48-Ohm
DWC_D5MPL2_ODTOFF   LPDDR2 DWC_D5M_PDDRIO cell ODT off Receiver
DWC_D5MPL3_34   LPDDR3 DWC_D5M_PDDRIO Supply-reminated cell  Z0=34-Ohm
DWC_D5MPL3_34M   LPDDR3 DWC_D5M_PDDRIO Mid-rail terminated cell  Z0=34-Ohm
DWC_D5MPL3_34ODT120   LPDDR3 DWC_D5M_PDDRIO cell ODT 120 Ohms Receiver
DWC_D5MPL3_34ODT240   LPDDR3 DWC_D5M_PDDRIO cell ODT 240 Ohms Receiver
DWC_D5MPL3_34ODT60   LPDDR3 DWC_D5M_PDDRIO Supply-terminated cell ODT 60 Ohms Receiver
DWC_D5MPL3_34ODTOFF   LPDDR3 DWC_D5M_PDDRIO cell ODT off Receiver
DWC_D5MPL3_40   LPDDR3 DWC_D5M_PDDRIO Supply-terminated cell  Z0=40-Ohm
DWC_D5MPL3_48   LPDDR3 DWC_D5M_PDDRIO Supply-terminated cell  Z0=48-Ohm
DWC_D5MPL3_48M   LPDDR3 DWC_D5M_PDDRIO Mid-rail terminated cell  Z0=48-Ohm
DWC_D5MPL3_ODT120M   LPDDR3 DWC_D5M_PDDRIO cell ODT 120 Ohms Receiver
DWC_D5MPL3_ODT240M   LPDDR3 DWC_D5M_PDDRIO cell ODT 240 Ohms Receiver
DWC_D5MPL4_40   LPDDR4 DWC_D5M_PDDRIO cell  Z0=40-Ohm Driver SR=00
DWC_D5MPL4_40_TXM   LPDDR4 DWC_D5M_PDDRIO cell  Z0=40-Ohm Driver SR=11 Pre-emphasis ON
DWC_D5MPL4_48   LPDDR4 DWC_D5M_PDDRIO cell  Z0=48-Ohm Driver SR=00
DWC_D5MPL4_48_TXM   LPDDR4 DWC_D5M_PDDRIO cell  Z0=48-Ohm Driver SR=11 Pre-emphasis ON
DWC_D5MPL4_60   LPDDR4 DWC_D5M_PDDRIO cell  Z0=60-Ohm Driver SR=00
DWC_D5MPL4_60_TXM   LPDDR4 DWC_D5M_PDDRIO cell  Z0=60-Ohm Driver SR=11 Pre-emphasis ON
DWC_D5MPL4_80   LPDDR4 DWC_D5M_PDDRIO cell  Z0=80-Ohm Driver SR=00
DWC_D5MPL4_80_TXM   LPDDR4 DWC_D5M_PDDRIO cell  Z0=80-Ohm Driver SR=11 Pre-emphasis ON
DWC_D5MPL4_ODT40   LPDDR4 DWC_D5M_PDDRIO cell 40-Ohm ODT Receiver
DWC_D5MPL4_ODT48   LPDDR4 DWC_D5M_PDDRIO cell 48-Ohm ODT Receiver
DWC_D5MPL4_ODT60   LPDDR4 DWC_D5M_PDDRIO cell 60-Ohm ODT Receiver
DWC_D5MPL4_ODT80   LPDDR4 DWC_D5M_PDDRIO cell 80-Ohm ODT Receiver
DWC_D5MPL4_ODTOFF   LPDDR4 DWC_D5M_PDDRIO cell  ODT off Receiver
[Model Selector] PDDRIO_PAD_DATA
DWC_D5MP3L_34   DDR3L DWC_D5M_PDDRIO cell  Z0=34-Ohm
DWC_D5MP3L_40   DDR3L DWC_D5M_PDDRIO cell  Z0=40-Ohm
DWC_D5MP3L_48   DDR3L DWC_D5M_PDDRIO cell  Z0=48-Ohm
DWC_D5MP3L_60   DDR3L DWC_D5M_PDDRIO cell  Z0=60-Ohm Driver SR=00
DWC_D5MP3L_60_TXM   DDR3L DWC_D5M_PDDRIO cell  Z0=60-Ohm Driver SR=11 Pre-emphasis ON
DWC_D5MP3L_ODT40   DDR3L DWC_D5M_PDDRIO cell 40-Ohm ODT Receiver
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| Models and submodels in the file (237): BDPROGSCARUDQP_SDMMC_3V3SF_00_MMC (I/O), BDPROGSCARUDQP_SDMMC_3V3SF_00_SD (I/O), BDPROGSCARUDQP_SDMMC_3V3SF_01_MMC (I/O), BDPROGSCARUDQP_SDMMC_3V3SF_01_SD (I/O), BDPROGSCARUDQP_SDMMC_3V3SF_10 (I/O), BDPROGSCARUDQP_SDMMC_3V3SF_10_2v7 (I/O), BDPROGSCARUDQP_SDMMC_3V3SF_11 (I/O), BDPROGSCARUDQP_SDMMC_3V3SF_11_2v7 (I/O), BDPROG_1V2_000 (I/O), BDPROG_1V2_001 (I/O), BDPROG_1V2_010 (I/O), BDPROG_1V2_011 (I/O), BDPROG_1V2_100 (I/O), BDPROG_1V2_101 (I/O), BDPROG_1V2_110 (I/O), BDPROG_1V2_111 (I/O), BDPROG_1V8_000 (I/O), BDPROG_1V8_001 (I/O), BDPROG_1V8_010 (I/O), BDPROG_1V8_011 (I/O), BDPROG_1V8_100 (I/O), BDPROG_1V8_101 (I/O), BDPROG_1V8_110 (I/O), BDPROG_1V8_111 (I/O), DWC_D5MC3L_34 (I/O), DWC_D5MC3L_40 (I/O), DWC_D5MC3L_48 (I/O), DWC_D5MC3L_ODT40 (Input), DWC_D5MC3L_ODT60 (Input), DWC_D5MC3L_ODTOFF (Input), DWC_D5MC3_34 (I/O), DWC_D5MC3_40 (I/O), DWC_D5MC3_48 (I/O), DWC_D5MC3_ODT40 (Input), DWC_D5MC3_ODT60 (Input), DWC_D5MC3_ODTOFF (Input), DWC_D5MC4_34 (I/O), DWC_D5MC4_34M (I/O), DWC_D5MC4_34M_TXM (I/O), DWC_D5MC4_34ODT40 (Input), DWC_D5MC4_34ODTOFF (Input), DWC_D5MC4_34_TXM (I/O), DWC_D5MC4_48 (I/O), DWC_D5MC4_48M (I/O), DWC_D5MC4_48M_TXM (I/O), DWC_D5MC4_48ODT60 (Input), DWC_D5MC4_48_TXM (I/O), DWC_D5MCK3L_34 (I/O), DWC_D5MCK3L_40 (I/O), DWC_D5MCK3L_48 (I/O), DWC_D5MCK3L_ODT40 (Input), DWC_D5MCK3L_ODT60 (Input), DWC_D5MCK3L_ODTOFF (Input), DWC_D5MCK3_34 (I/O), DWC_D5MCK3_40 (I/O), DWC_D5MCK3_48 (I/O), DWC_D5MCK3_ODT40 (Input), DWC_D5MCK3_ODT60 (Input), DWC_D5MCK3_ODTOFF (Input), DWC_D5MCK4_34 (I/O), DWC_D5MCK4_34M (I/O), DWC_D5MCK4_34M_TXM (I/O), DWC_D5MCK4_34ODT40 (Input), DWC_D5MCK4_34ODTOFF (Input), DWC_D5MCK4_34_TXM (I/O), DWC_D5MCK4_48 (I/O), DWC_D5MCK4_48M (I/O), DWC_D5MCK4_48M_TXM (I/O), DWC_D5MCK4_48ODT60 (Input), DWC_D5MCK4_48_TXM (I/O), DWC_D5MCKL2_34 (I/O), DWC_D5MCKL2_48 (I/O), DWC_D5MCKL2_ODTOFF (Input), DWC_D5MCKL3_34 (I/O), DWC_D5MCKL3_34M (I/O), DWC_D5MCKL3_34ODT120 (Input), DWC_D5MCKL3_34ODT240 (Input), DWC_D5MCKL3_34ODT60 (Input), DWC_D5MCKL3_34ODTOFF (Input), DWC_D5MCKL3_40 (I/O)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
